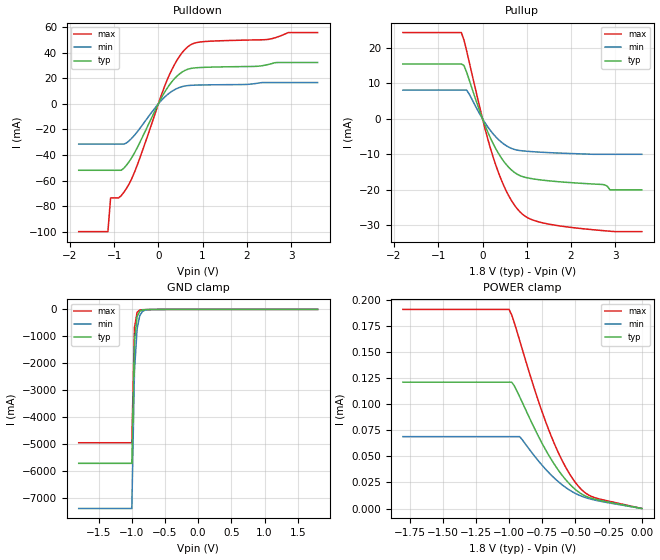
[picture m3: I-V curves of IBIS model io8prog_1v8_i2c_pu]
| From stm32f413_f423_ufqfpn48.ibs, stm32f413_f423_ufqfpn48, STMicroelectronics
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[Model]  io8prog_1v8_i2c_pu
Model_type I/O
Polarity   Non-Inverting
Enable   Active-Low
Vinl =   0.540000V
Vinh =   1.260000V
Vmeas =  0.900000V
Cref =   100.000000pF
Rref =   1.000000k
Vref =   1.800000V
C_comp   2.500900pF   2.333900pF   2.735800pF
[Temperature Range]   25.000000   0.125000k   -40.000000
[Pullup Reference]   1.800000V   1.600000V   2.000000V
[Pulldown Reference]   0.0V   0.0V   0.0V
[POWER Clamp Reference]   1.800000V   1.600000V   2.000000V
[GND Clamp Reference]   0.0V   0.0V   0.0V
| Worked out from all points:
|   slope of the pulldown table from 0 to 0.27 V, typ, clamps not added: 17.2 ohm
|   slope of the pullup table from 0 to 0.27 V, typ, clamps not added: 34.9 ohm
|   GND clamp passes 1 mA (typ) near -0.57 V on its own axis
[Pulldown]
|Voltage   I(typ)   I(min)   I(max)
-1.8V     -51.99mA   -31.53mA   -100mA
-1.14V    -51.99mA   -31.53mA   -100mA
-1.08V    -51.99mA   -31.53mA   -73.63mA
-900mV    -51.99mA   -31.53mA   -73.63mA
-660mV    -45.19mA   -28.93mA   -62.58mA
-480mV    -34.51mA   -22.06mA   -48.23mA
240mV     14.31mA    8.182mA    21.95mA
480mV     23.44mA    12.84mA    37.31mA
660mV     26.99mA    14.27mA    44.47mA
960mV     28.44mA    14.75mA    48.45mA
2.46V     30.59mA    16.64mA    50.31mA
3.6V      32.32mA    16.64mA    55.78mA
[Pullup]
|Voltage   I(typ)   I(min)   I(max)
-1.8V     15.46mA    8.102mA    24.33mA
-480mV    15.46mA    8.102mA    24.33mA
-360mV    13.15mA    8.102mA    19.18mA
60mV      -1.95mA    -1.198mA   -2.977mA
300mV     -8.441mA   -5.092mA   -13.07mA
600mV     -13.78mA   -8.025mA   -21.88mA
900mV     -16.27mA   -9.02mA    -26.86mA
1.2V      -17.03mA   -9.318mA   -28.8mA
1.74V     -17.74mA   -9.658mA   -30.18mA
2.76V     -18.6mA    -10mA      -31.55mA
2.88V     -20mA      -10mA      -31.68mA
3.6V      -20mA      -10mA      -31.8mA
[GND_clamp]
|Voltage   I(typ)   I(min)   I(max)
-1.8V     -5.722A    -7.401A    -4.956A
-1V       -5.722A    -7.401A    -4.956A
-960mV    -1.203A    -2.294A    -680.3mA
-920mV    -260.8mA   -717.4mA   -103.7mA
-880mV    -62.26mA   -228.9mA   -23.84mA
-840mV    -19.05mA   -76.32mA   -11.31mA
-760mV    -5.573mA   -11.66mA   -6.2mA
-640mV    -2.048mA   -2.413mA   -2.197mA
1.8V      0A         0A         0A
[POWER_clamp]
|Voltage   I(typ)   I(min)   I(max)
-1.8V     121uA      68.85uA    190.7uA
-1V       121uA      68.85uA    190.7uA
-980mV    121uA      68.85uA    185.3uA
-960mV    117.4uA    68.85uA    177.7uA
-920mV    107uA      68.85uA    160.9uA
-800mV    74.53uA    48.91uA    111uA
-720mV    55.17uA    36.99uA    81.65uA
-620mV    35.16uA    24.73uA    51.11uA
-520mV    20.42uA    15.79uA    28.41uA
-440mV    12.93uA    11.16uA    16.44uA
-380mV    9.841uA    8.86uA     11.63uA
0V        0A         11.08nA    0A
[Ramp]
| variable   typ   min   max
dV/dt_r  0.49600/6.00000u   0.27832/6.00000u   0.74721/6.00000u
dV/dt_f  0.75169/6.00000u   0.43965/6.00000u   0.96654/6.00000u
R_load = 50.000000
